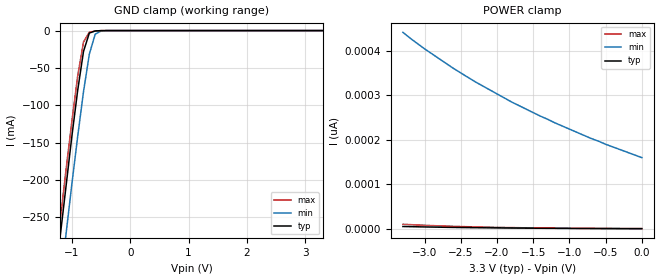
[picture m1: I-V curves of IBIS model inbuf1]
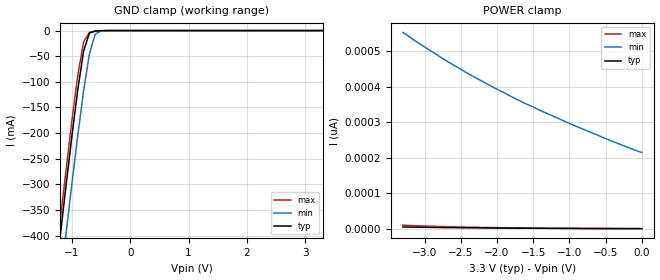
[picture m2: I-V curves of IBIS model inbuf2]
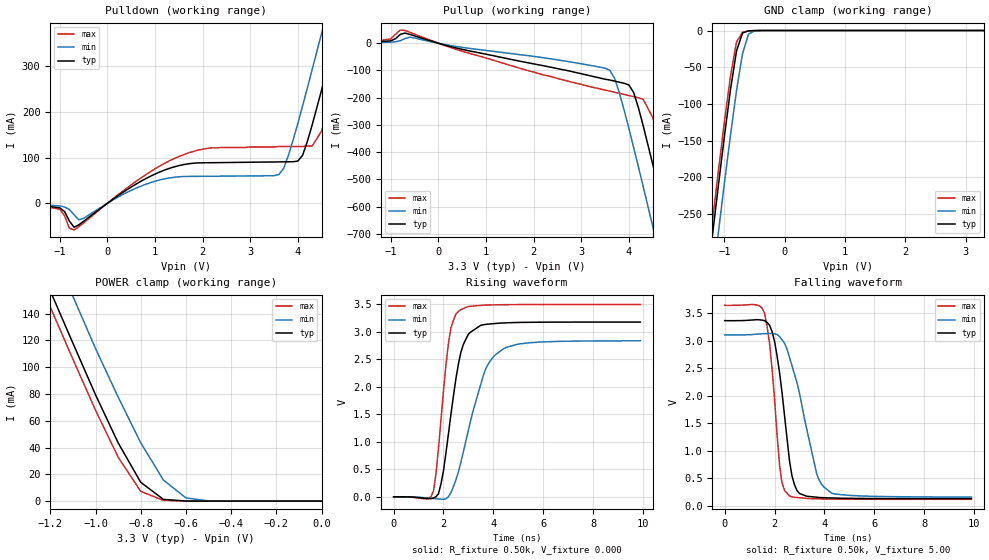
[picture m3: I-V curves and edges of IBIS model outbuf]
| IBIS file 63374l.ibs created by s2ibis2 version 1.0
| North Carolina State University Electronics Research Laboratory  1995
[IBIS ver]   2.1
[File name]   63374l.ibs
[File Rev]   0.1
[Date]   Monday, June 2, 1997
[Source]   IDT
[Notes]   1. Temp typ=25C, min=100C, max=0C 2. Ramp rates based on 500
   ohm load
[Copyright]   Copyright 1997, Integrated Device Technology, Inc.
[Disclaimer] Integrated Device Technology, Inc. ("IDT") hereby grants the
   user of this IBIS model a non-exclusive, nontransferable
   license to use this IBIS model under the following terms.
   The user is granted this license only to use the IBIS model
   and is not granted rights to sell, copy (except as needed to
   run the IBIS model), rent, lease or sub-license the IBIS model
   in whole or in part, or in modified form to anyone.
   The User may modify the IBIS model to suit its specific
   applications, but rights to derivative works and such
   modifications shall belong to IDT.
   This IBIS model is provided on an "AS IS" basis and IDT
   makes absolutely no warranty with respect to the information
   contained herein. IDT DISCLAIMS AND CUSTOMER WAIVES ALL
   WARRANTIES, EXPRESS AND IMPLIED, INCLUDING WARRANTIES OF
   MERCHANTABILITY AND FITNESS FOR A PARTICULAR PURPOSE. THE
   ENTIRE RISK AS TO QUALITY AND PERFORMANCE IS WITH THE
   USER ACCORDINGLY, IN NO EVENT SHALL IDT BE LIABLE
   FOR ANY DIRECT OR INDIRECT DAMAGES, WHETHER IN CONTRACT OR
   TORT, INCLUDING ANY LOST PROFITS OR OTHER INCIDENTAL,
   CONSEQUENTIAL, EXEMPLARY, OR PUNITIVE DAMAGES ARISING OUT OF
   THE USE OR APPLICATION OF THE IBIS model.  Further, IDT
   reserves the right to make changes without notice to any
   product herein to improve reliability, function, or design.
   IDT does not convey any license under patent rights or
   any other intellectual property rights, including those of
   third parties. IDT is not obligated to provide maintenance
   or support for the licensed IBIS model.
|   Component IDT54/74FCT163374/A/C
[Component]   IDT54/74FCT163374/A/C
[Manufacturer]   Integrated Device Technology Inc.
[Package]
| Following package parameters are for SO48-2(TSSOP) package
|[Package]
|| variable   typ   min   max
|R_pkg   15.00m   10.00m   20.00m
|L_pkg   2.30nh   1.40nh   4.50nH
|C_pkg   0.40pF   0.35pF   0.60pF
| Following package parameters are for SO48-1(SSOP), E48-1(CERPAK) packages
| variable   typ   min   max
R_pkg   15.00m   10.00m   20.00m
L_pkg   2.90nH   1.50nH   5.60nH
C_pkg   0.40pF   0.26pF   0.50pF
[Pin]  signal_name   model_name   R_pin   L_pin   C_pin
1   1OEB   inbuf1
2   1O1   outbuf
3   1O2   outbuf
4   GND   GND
5   1O3   outbuf
6   1O4   outbuf
7   VCC   POWER
8   1O5   outbuf
9   1O6   outbuf
10   GND   GND
11   1O7   outbuf
12   1O8   outbuf
13   2O1   outbuf
14   2O2   outbuf
15   GND   GND
16   2O3   outbuf
17   2O4   outbuf
18   VCC   POWER
19   2O5   outbuf
20   2O6   outbuf
21   GND   GND
22   2O7   outbuf
23   2O8   outbuf
24   2OEB   inbuf1
25   2CLK   inbuf1
26   2D8   inbuf2
27   2D7   inbuf2
28   GND   GND
29   2D6   inbuf2
30   2D5   inbuf2
31   VCC   POWER
32   2D4   inbuf2
33   2D3   inbuf2
34   GND   GND
35   2D2   inbuf2
36   2D1   inbuf2
37   1D8   inbuf2
38   1D7   inbuf2
39   GND   GND
40   1D6   inbuf2
41   1D5   inbuf2
42   VCC   POWER
43   1D4   inbuf2
44   1D3   inbuf2
45   GND   GND
46   1D2   inbuf2
47   1D1   inbuf2
48   1CLK   inbuf1
| Models and submodels in the file (3): inbuf1 (Input), inbuf2 (Input), outbuf (3-state)
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| in   IN1   dummy_model
| oe   OE1   dummy_model
|   Model inbuf1
[Model]   inbuf1
Model_type   Input
Vinl =  0.800V
Vinh =  2.000V
C_comp   3.00pF   NA   NA
[Temperature Range]   25.00   100.00   0.000
[Voltage Range]   3.30V   3.00V   3.60V
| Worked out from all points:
|   GND clamp passes 1 mA (typ) near -0.62 V on its own axis
[GND_clamp]
| voltage   I(typ)   I(min)   I(max)
-3.3V     -1.781A    -1.841A    -1.762A
-1.3V     -346mA     -410mA     -324mA
-1.2V     -276mA     -341mA     -255mA
-1.1V     -209mA     -273mA     -187mA
-1V       -142mA     -206mA     -122mA
-900mV    -80.26mA   -142mA     -61.07mA
-800mV    -27.87mA   -81.82mA   -15.26mA
-700mV    -3.289mA   -31.47mA   -2.24mA
-600mV    -480uA     -4.848mA   -551uA
-500mV    -82.77uA   -464uA     -85.69uA
3.3V      588fA      178pA      482fA
[POWER_clamp]
| voltage   I(typ)   I(min)   I(max)
-3.3V     5.432pA    441pA      10.51pA
-3V       4.444pA    404pA      8.155pA
-2.6V     3.398pA    360pA      5.808pA
-2.3V     2.779pA    330pA      4.5pA
-1.8V     1.984pA    285pA      2.938pA
-1.2V     1.325pA    238pA      1.756pA
-700mV    945fA      203pA      1.142pA
0V        588fA      160pA      625fA
|   Model inbuf2
[Model]   inbuf2
Model_type   Input
Vinl =  0.800V
Vinh =  2.000V
C_comp   3.00pF   NA   NA
[Temperature Range]   25.00   100.00   0.000
[Voltage Range]   3.30V   3.00V   3.60V
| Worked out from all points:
|   GND clamp passes 1 mA (typ) near -0.60 V on its own axis
[GND_clamp]
| voltage   I(typ)   I(min)   I(max)
-3.3V     -2.589A    -2.677A    -2.561A
-1.3V     -502mA     -596mA     -472mA
-1.2V     -402mA     -496mA     -371mA
-1.1V     -303mA     -397mA     -273mA
-1V       -207mA     -300mA     -177mA
-900mV    -117mA     -206mA     -88.94mA
-800mV    -40.68mA   -119mA     -22.5mA
-700mV    -5.011mA   -45.86mA   -3.669mA
-600mV    -847uA     -7.149mA   -1.066mA
-500mV    -175uA     -726uA     -214uA
3.3V      678fA      238pA      568fA
[POWER_clamp]
| voltage   I(typ)   I(min)   I(max)
-3.3V     5.52pA     553pA      10.45pA
-3.1V     4.852pA    525pA      8.856pA
-2.7V     3.752pA    473pA      6.363pA
-2.4V     3.095pA    437pA      4.968pA
-1.8V     2.111pA    372pA      3.038pA
-1.4V     1.639pA    333pA      2.195pA
-900mV    1.196pA    288pA      1.468pA
-500mV    931fA      254pA      1.067pA
0V        678fA      215pA      718fA
|   Model outbuf
[Model]   outbuf
Model_type   3-state
Polarity   Non-Inverting
Enable   Active-High
Vinl =  0.800V
Vinh =  2.000V
C_comp   3.00pF   NA   NA
[Temperature Range]   25.00   100.00   0.000
[Voltage Range]   3.30V   3.00V   3.60V
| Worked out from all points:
|   slope of the pulldown table from 0 to 0.495 V, typ, clamps not added: 14.1 ohm
|   slope of the pullup table from 0 to 0.495 V, typ, clamps not added: 22.2 ohm
|   GND clamp passes 1 mA (typ) near -0.62 V on its own axis
|   POWER clamp passes 1 mA (typ) near -0.67 V on its own axis
|   rising waveform, R_fixture 0.50k, V_fixture 0.000: 20-80 % time 609ps typ, 986ps min, 442ps max; typ from 0 V to 3.17 V
|   falling waveform, R_fixture 0.50k, V_fixture 5.00: 20-80 % time 512ps typ, 891ps min, 384ps max; typ from 3.36 V to 0.129 V
[Pulldown]
| voltage   I(typ)   I(min)   I(max)
-3.3V     -1mA       0A         -1mA
-1V       -10.1mA    -5.8mA     -13.1mA
-700mV    -52.41mA   -25.02mA   -58.28mA
1.5V      82.23mA    57.84mA    102mA
3.6V      90.38mA    62.61mA    124mA
3.8V      90.63mA    104mA      124mA
4.1V      105mA      213mA      124mA
4.3V      171mA      292mA      125mA
4.5V      248mA      372mA      158mA
4.9V      411mA      535mA      311mA
5.1V      494mA      618mA      393mA
6.6V      1.122A     1.24A      1.022A
[Pullup]
| voltage   I(typ)   I(min)   I(max)
-3.3V     0A         1mA        1mA
-1.5V     2.3mA      1.4mA      3mA
-700mV    37.47mA    17.46mA    46.94mA
3.5V      -132mA     -91.52mA   -172mA
3.7V      -139mA     -129mA     -180mA
4.1V      -181mA     -383mA     -196mA
4.3V      -303mA     -526mA     -206mA
4.5V      -444mA     -672mA     -272mA
4.7V      -590mA     -820mA     -406mA
4.9V      -738mA     -968mA     -551mA
5.1V      -887mA     -1.116A    -698mA
6.6V      -2.019A    -2.242A    -1.829A
[GND_clamp]
| voltage   I(typ)   I(min)   I(max)
-3.3V     -1.845A    -1.891A    -1.839A
-1.3V     -351mA     -414mA     -332mA
-1.2V     -280mA     -344mA     -261mA
-1.1V     -211mA     -275mA     -191mA
-1V       -144mA     -208mA     -124mA
-900mV    -80.93mA   -143mA     -62.38mA
-800mV    -28.09mA   -82.05mA   -15.75mA
-700mV    -3.331mA   -31.56mA   -2.343mA
-600mV    -482uA     -4.864mA   -563uA
-500mV    -82.6uA    -465uA     -86.04uA
3.3V      639fA      360nA      501fA
[POWER_clamp]
| voltage   I(typ)   I(min)   I(max)
-3.3V     1.028A     1.052A     1.02A
-1.3V     197mA      231mA      185mA
-1.2V     157mA      192mA      145mA
-1.1V     118mA      153mA      106mA
-1V       79.45mA    114mA      67.95mA
-900mV    43.56mA    77.76mA    32.88mA
-800mV    14.07mA    43.59mA    7.263mA
-700mV    1.334mA    15.8mA     596uA
-600mV    60.43uA    2.386mA    67.13uA
-500mV    2.01uA     169uA      3.696uA
0V        639fA      159pA      682fA
[Ramp]
| variable   typ   min   max
dV/dt_r   1.90/0.61n   1.70/0.99n   2.09/0.44n
dV/dt_f   1.93/0.52n   1.74/0.81n   2.11/0.39n
R_load = 0.50k
[Rising Waveform]
R_fixture = 0.50k
V_fixture = 0.000
| time   V(typ)   V(min)   V(max)
0s        0V         0V         0V
1.6ns     -20.72mV   -29.7mV    106mV
1.9ns     237mV      -42.26mV   1.404V
2.2ns     1.15V      1.166mV    2.789V
2.3ns     1.502V     77.53mV    3.068V
2.6ns     2.412V     456mV      3.365V
3ns       2.955V     1.211V     3.453V
3.7ns     3.13V      2.329V     3.481V
4.4ns     3.156V     2.684V     3.487V
9.9ns     3.172V     2.832V     3.491V
[Falling Waveform]
R_fixture = 0.50k
V_fixture = 5.00
| time   V(typ)   V(min)   V(max)
0s        3.363V     3.103V     3.641V
1.6ns     3.362V     3.126V     3.496V
1.9ns     3.166V     3.129V     2.491V
2.2ns     2.422V     3.072V     746mV
2.3ns     2.059V     3.013V     421mV
2.6ns     817mV      2.695V     179mV
2.9ns     276mV      2.238V     149mV
3.7ns     154mV      564mV      125mV
4.3ns     141mV      227mV      120mV
9.9ns     129mV      158mV      116mV
